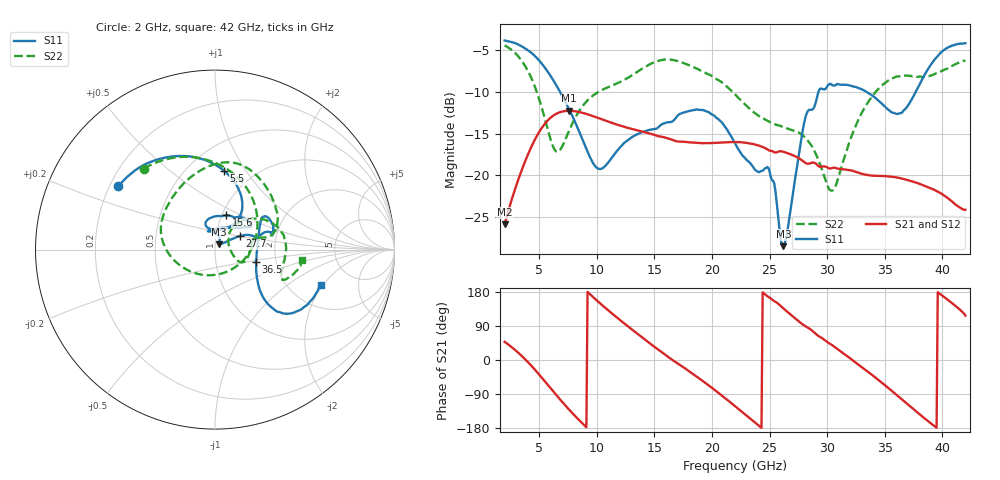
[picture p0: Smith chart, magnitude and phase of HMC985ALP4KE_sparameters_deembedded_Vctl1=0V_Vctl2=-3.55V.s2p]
!s2p File: Measurements: S11, S21, S12, S22
# GHz S dB R 50.0
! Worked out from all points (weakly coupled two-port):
!   401 points, 2 GHz to 42 GHz, reference 50 ohm
!   highest |S21| = -12.27 dB at 7.6 GHz (marker M1); lowest = -25.9 dB at 2 GHz (marker M2)
!   lowest |S11| = -28.5 dB at 26.2 GHz (marker M3), VSWR 1.08, Z = 52.3 + j3.09 ohm
!   |S11| at or under -10 dB: 6.813 GHz to 29.25 GHz (22.44 GHz wide, 124 % of centre); 33.41 GHz to 37.69 GHz (4.279 GHz wide, 12 % of centre)
!   |S22| runs from -21.8 to -4.4 dB; largest |S21 - S12| = 0.00033
!   S11 on the Smith chart (normalised r, x): 2 GHz: 0.23, +0.28; 5.5 GHz: 0.74, +0.80; 15.6 GHz: 1.05, +0.42; 27.7 GHz: 1.30, +0.20; 36.5 GHz: 1.57, -0.23; 42 GHz: 2.94, -1.89
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2  -3.83 146.8  -25.90 48.0  -25.90 48.0  -4.42 131.3
3.6  -4.62 119.9  -18.97 7.4  -18.97 7.4  -6.51 86.9
5.5  -7.11 83.3  -13.81 -56.5  -13.82 -56.5  -13.26 8.0
6.5  -9.23 66.1  -12.61 -92.9  -12.60 -93.0  -17.15 -67.1
7.6  -12.08 54.2  -12.27 -131.0  -12.27 -131.0  -14.64 -139.8
8.7  -15.50 54.6  -12.48 -165.6  -12.48 -165.7  -11.82 -174.0
10.3  -19.25 88.1  -13.22 149.2  -13.20 149.2  -9.88 160.1
12.6  -15.89 109.0  -14.28 91.4  -14.27 91.4  -8.38 126.6
15.4  -14.17 75.5  -15.33 26.1  -15.34 26.1  -6.24 84.6
15.6  -13.92 71.8  -15.37 21.7  -15.38 21.6  -6.18 82.2
19.3  -12.21 33.5  -16.14 -57.5  -16.14 -57.5  -7.60 36.6
22  -16.14 51.5  -16.01 -121.8  -16.01 -121.8  -10.29 13.6
24.9  -19.09 104.4  -16.98 166.4  -16.96 166.4  -13.52 11.7
26.2  -28.51 51.8  -17.18 136.2  -17.19 136.2  -14.22 -4.1
27.7  -16.15 28.7  -18.09 98.0  -18.11 97.9  -15.04 -22.3
28.7  -12.13 12.7  -18.49 77.3  -18.48 77.3  -16.56 -26.5
30.5  -9.22 18.3  -19.11 37.7  -19.11 37.7  -21.80 19.6
32.9  -9.63 34.0  -19.78 -16.7  -19.78 -16.7  -12.79 45.7
35.4  -12.22 11.7  -20.14 -76.2  -20.14 -76.2  -8.57 18.7
36.5  -12.48 -16.6  -20.40 -104.3  -20.40 -104.3  -8.05 6.1
39.5  -5.85 -43.6  -21.89 -178.8  -21.89 -178.8  -7.75 -23.7
42  -4.15 -18.6  -24.14 117.1  -24.16 117.1  -6.20 -7.0
